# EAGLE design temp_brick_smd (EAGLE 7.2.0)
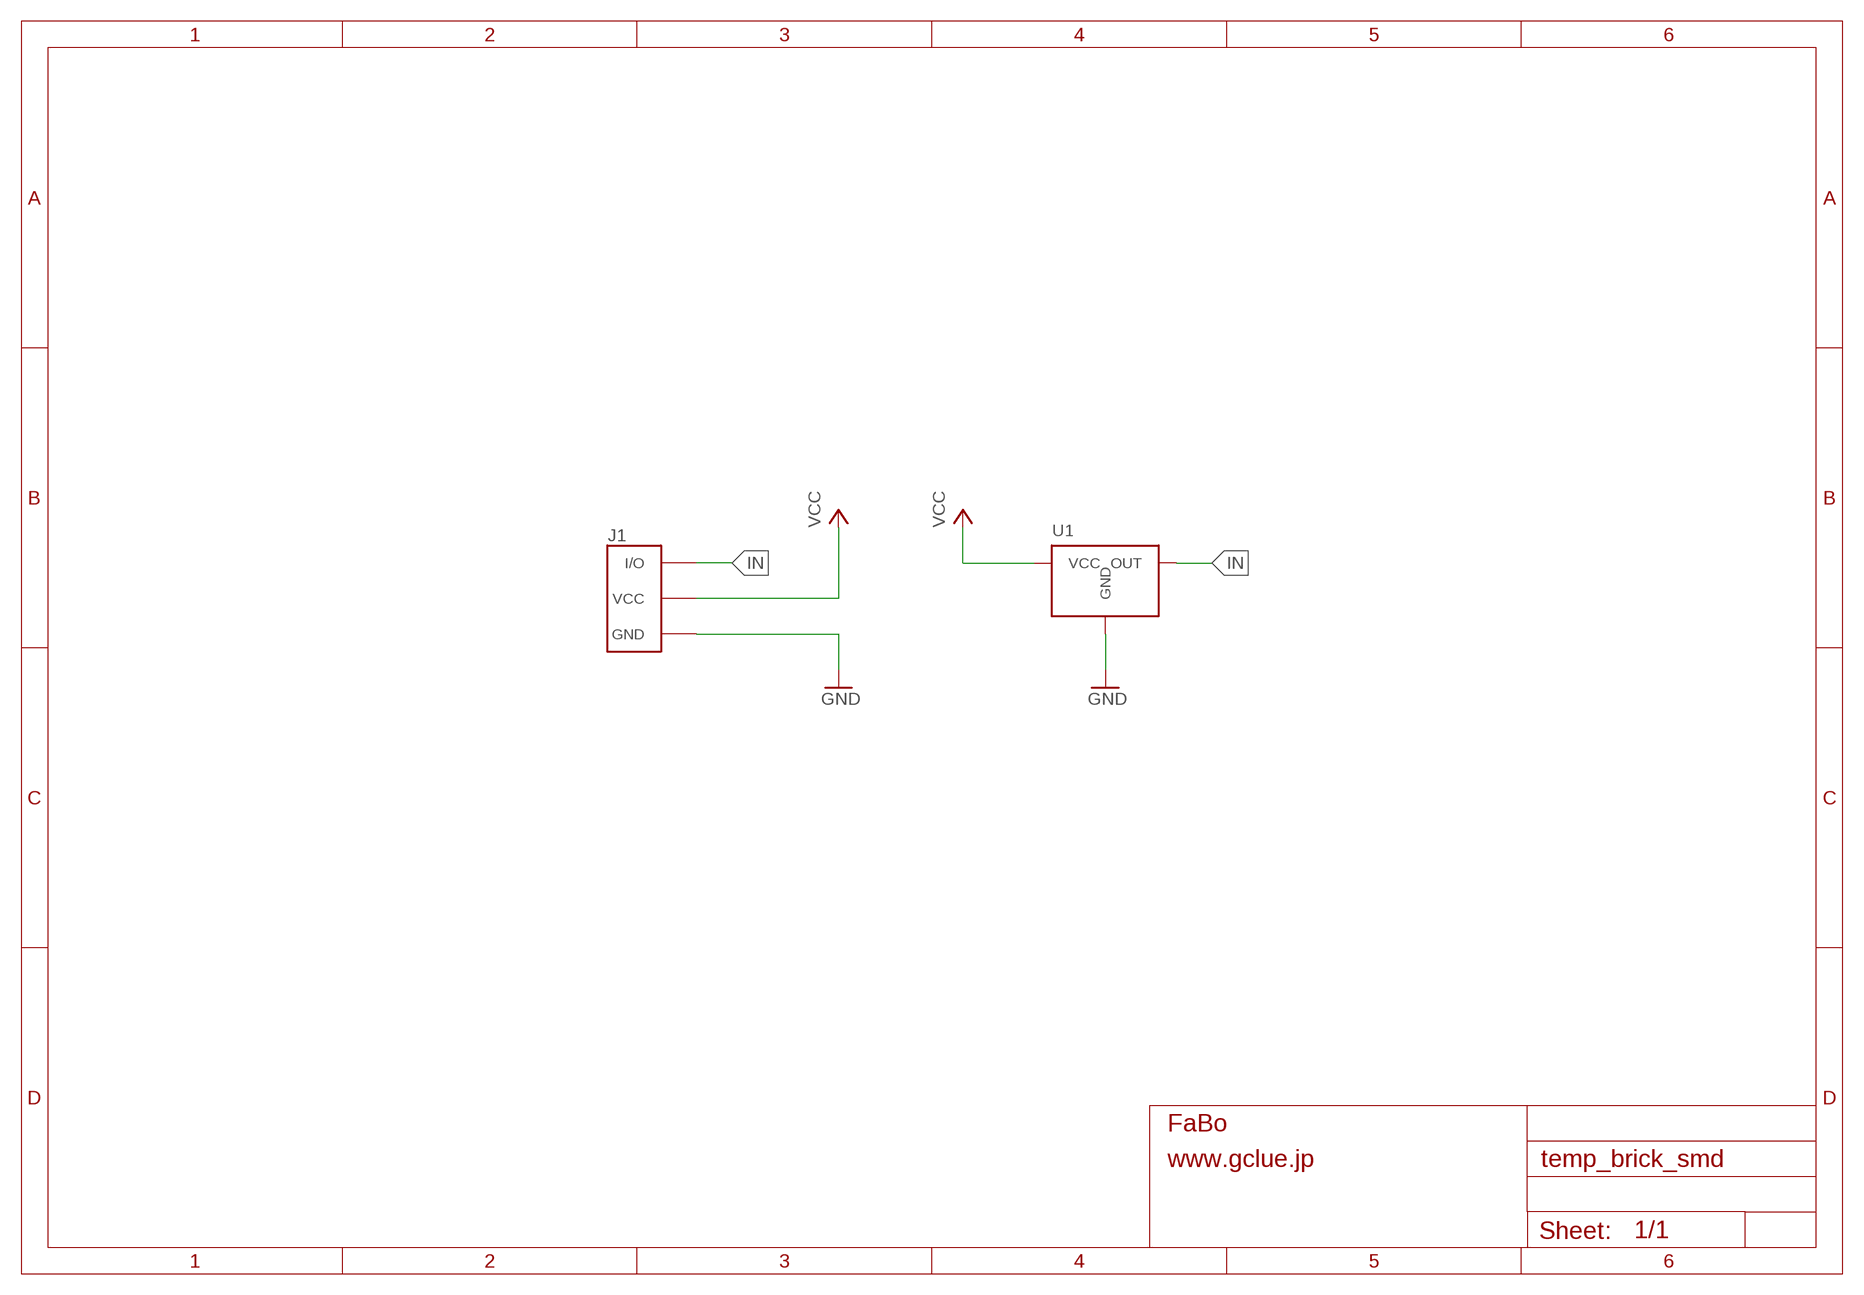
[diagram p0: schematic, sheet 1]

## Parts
J1  BRICK_3PIN  [BRICK_3PIN]
U1  SENSOR-LM60-SOT  [SENSOR-LM60-SOT-23]

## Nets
GND: J1.GND U1.GND
IN: J1.IN/OUT(I/O) U1.OUT
VCC: J1.VCC U1.VCC

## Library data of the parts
J1 = Gclue:BRICK_3PIN: FaBo Brick 3pin
U1 = Gclue:SENSOR-LM60-: LM60 Temperature Sensor

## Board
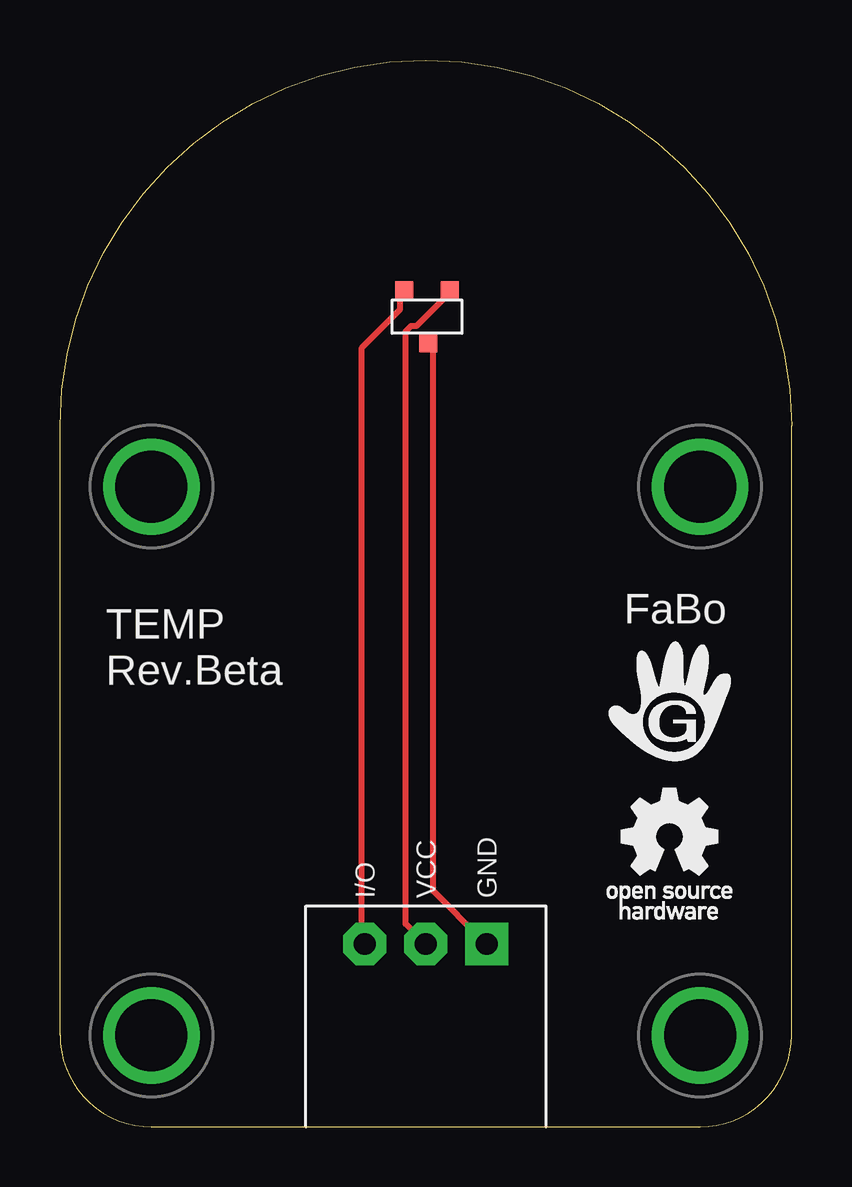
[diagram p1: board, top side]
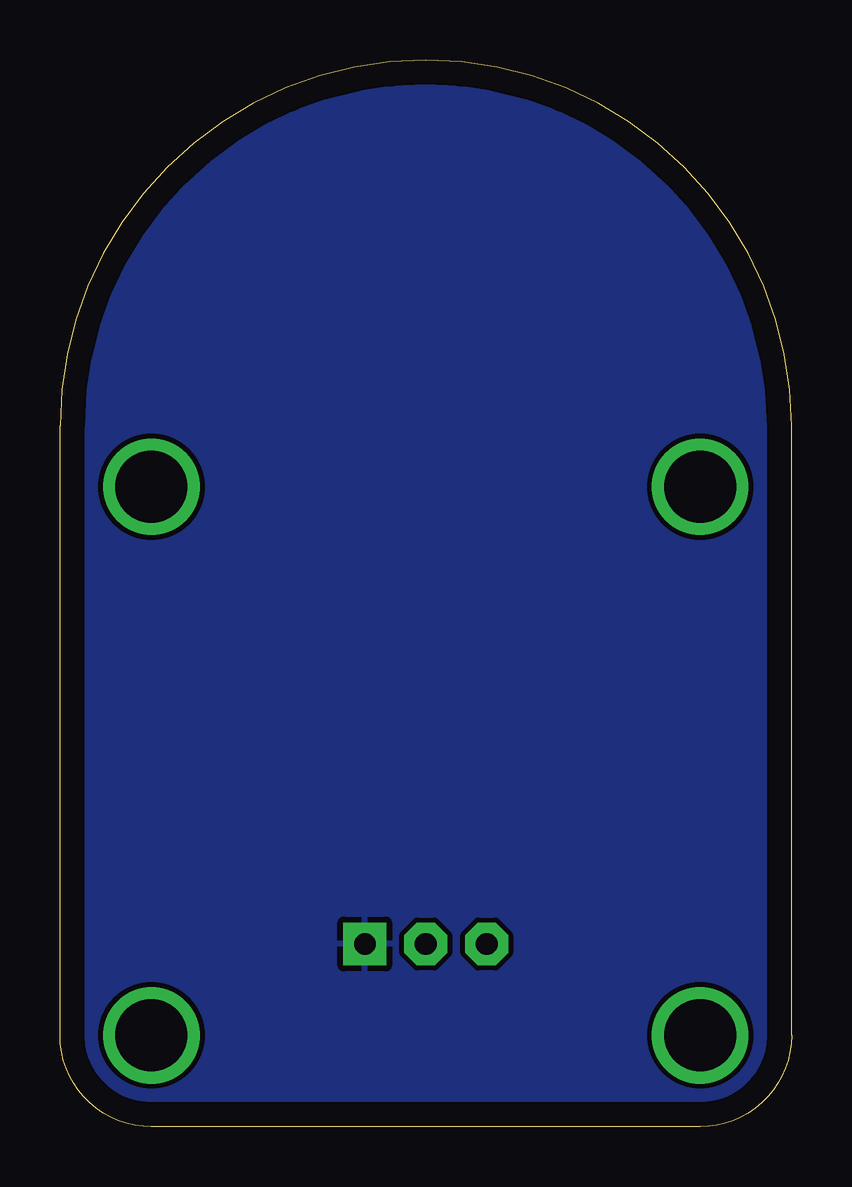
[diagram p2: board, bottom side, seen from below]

Size 30.48 x 44.45 mm. Coordinates in mm from the lower left corner, seen from the top.
Copper layers (1*16): Top 0.035mm / dielectric 1.5mm / Bottom 0.035mm
Design rules "default": minimum track width 10mil, minimum drill 24mil, track to track 8mil, track to pad 8mil, pad to pad 8mil, via to via 8mil, smd to smd 8mil, copper to edge 40mil, drill to drill 8mil, minimum pad ring 10mil, minimum via ring 8mil, stop-mask expansion 4mil, vias tented up to drill 0mil, thermal gap 10mil

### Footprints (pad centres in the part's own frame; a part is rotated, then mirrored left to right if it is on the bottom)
BRICK_3PIN = drill 0.9 pad 1.778 square: GND 2.54,-11.43 | drill 0.9 pad 1.778 octagon: IN/OUT -2.54,-11.43; VCC 0,-11.43 | drill 3 pad 3.81: P$1 -11.43,7.62; P$2 11.43,7.62; P$3 11.43,-15.24; P$4 -11.43,-15.24
SENSOR-LM60-SOT-23 = smd 0.76 x 0.76: GND -0.1,1; OUT 0.9,-1.2; VCC -1,-1.2

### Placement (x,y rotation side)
J1  15.24,19.05 0 top
U1  15.24,33.66 180 top
U$2  [LOGO_OSHW_T_M]  25.4,12.06 0 top
U$3  [LOGO_GCLUE_M]  25.4,17.78 0 top

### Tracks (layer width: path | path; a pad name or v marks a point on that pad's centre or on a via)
GND
  Top 0.254: U1.GND 15.54,32.46 15.54,9.83 17.6,7.77 J1.GND
  pour Bottom: 0,0 30.48,0 30.48,44.45 0,44.45
IN
  Top 0.254: U1.OUT 14.17,34.75 14.17,34.06 12.57,32.46 12.57,7.77 J1.IN/OUT
VCC
  Top 0.254: J1.VCC 14.4,8.46 14.4,33.15 14.63,33.38 14.86,33.38 16.23,34.75 U1.VCC

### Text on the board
tPlace: FaBo | TEMP / Rev.Beta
